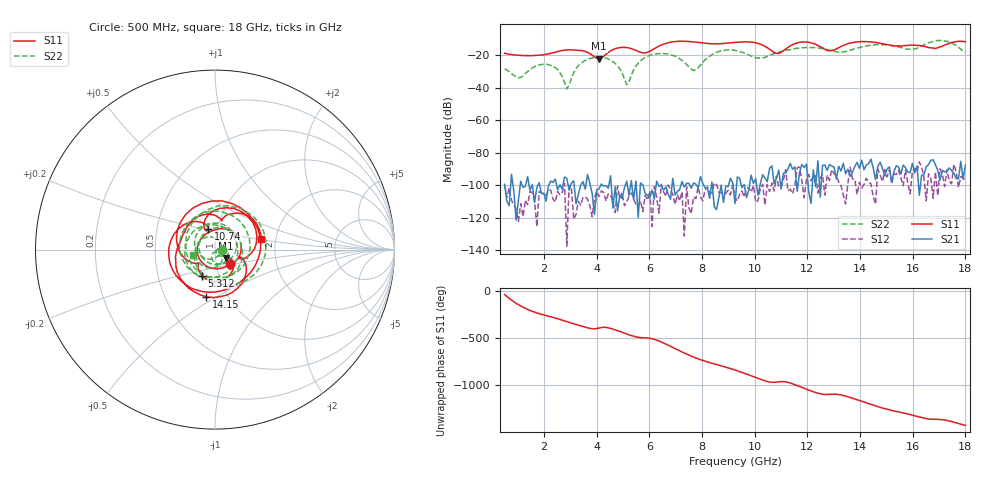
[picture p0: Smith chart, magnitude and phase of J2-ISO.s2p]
!Agilent Technologies,N5230A,MY45001360,A.07.50.67
!Agilent N5230A: A.07.50.67
!Date: Tuesday, April 16, 2024 15:50:35
!Correction: S11(Full 2 Port(1,2))
!S21(Full 2 Port(1,2))
!S12(Full 2 Port(1,2))
!S22(Full 2 Port(1,2))
!S2P File: Measurements: S11, S21, S12, S22:
# Hz S  dB  R 50
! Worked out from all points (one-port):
!   201 points, 500 MHz to 18 GHz, reference 50 ohm
!   lowest |S11| = -22.1 dB at 4.088 GHz (marker M1), VSWR 1.17, Z = 56.4 - j5.4 ohm
!   |S11| at or under -10 dB: start of sweep to end of sweep
!   S11 on the Smith chart (normalised r, x): 500 MHz: 1.17, -0.19; 5.312 GHz: 0.83, -0.25; 10.74 GHz: 0.90, +0.21; 14.15 GHz: 0.80, -0.45; 18 GHz: 1.68, +0.20
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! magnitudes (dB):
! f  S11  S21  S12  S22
! 500 MHz  -18.6  -99.5  -99.8  -28.4
! 1.113 GHz  -20.0  -97.7  -111.5  -33.7
! 2.25 GHz  -18.7  -97.5  -103.1  -26.2
! 2.862 GHz  -16.6  -95.8  -137.7  -40.7
! 3.475 GHz  -17.1  -97.9  -107.8  -24.0
! 4.088 GHz  -22.1  -102.4  -107.0  -21.0
! 4.787 GHz  -15.5  -116.0  -100.7  -26.4
! 5.138 GHz  -15.2  -97.6  -110.4  -38.1
! 5.312 GHz  -15.8  -97.2  -104.9  -32.2
! 5.75 GHz  -18.5  -99.9  -116.4  -22.2
! 6.362 GHz  -14.2  -100.8  -117.3  -18.8
! 7.675 GHz  -11.7  -98.7  -107.4  -29.2
! 8.463 GHz  -12.8  -113.3  -98.7  -18.7
! 9.25 GHz  -12.0  -111.5  -107.8  -16.9
! 10.74 GHz  -18.2  -99.2  -103.7  -18.9
! 12.22 GHz  -12.7  -90.6  -94.4  -15.1
! 12.84 GHz  -17.2  -87.3  -97.1  -16.6
! 14.15 GHz  -11.5  -90.5  -99.6  -14.4
! 15.11 GHz  -13.6  -88.7  -90.7  -13.7
! 15.99 GHz  -13.6  -86.6  -91.5  -16.2
! 17.12 GHz  -14.3  -90.9  -93.1  -10.8
! 18 GHz  -11.5  -87.8  -96.9  -17.9
